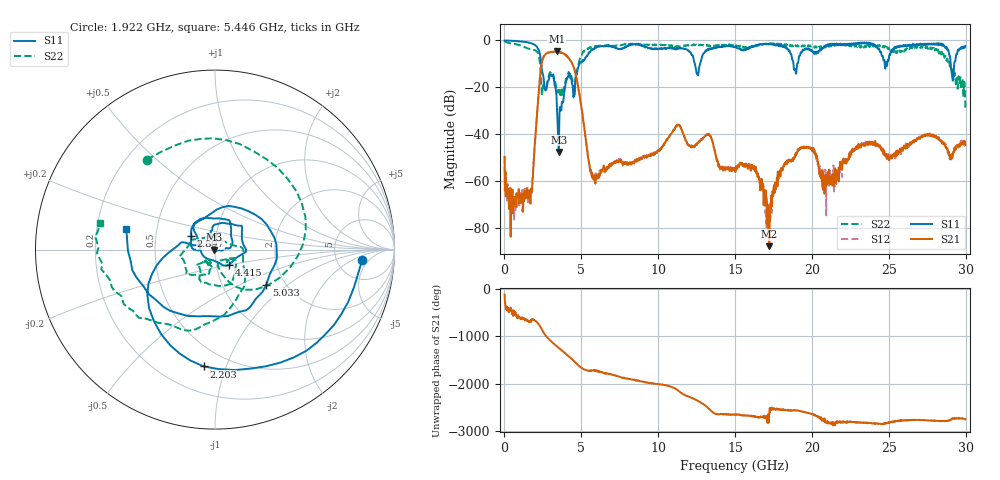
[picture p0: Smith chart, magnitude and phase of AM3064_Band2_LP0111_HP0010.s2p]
# Hz S DB R 50.0
!freq dBS11 angS11 dBS21 angS21 dBS12 angS12 dBS22 angS22
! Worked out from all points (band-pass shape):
!   1600 points, 10 MHz to 29.98 GHz, reference 50 ohm
!   highest |S21| = -4.74 dB at 3.403 GHz (marker M1); lowest = -87.9 dB at 17.22 GHz (marker M2)
!   |S21| within 3 dB of the highest: 2.503 GHz to 4.196 GHz (1.692 GHz wide, 50.5 % of centre)
!   lowest |S11| = -47.7 dB at 3.534 GHz (marker M3), VSWR 1.01, Z = 49.6 - j0.0628 ohm
!   |S11| at or under -10 dB: 2.398 GHz to 4.876 GHz (2.478 GHz wide, 68.1 % of centre); 12.38 GHz to 12.73 GHz (342.2 MHz wide, 2.73 % of centre); 18.8 GHz to 19.05 GHz (251.1 MHz wide, 1.33 % of centre)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
!   |S22| runs from -29.2 to -0.2 dB; largest |S21 - S12| = 0.016
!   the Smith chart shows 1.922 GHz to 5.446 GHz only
!   S11 on the Smith chart (normalised r, x): 1.922 GHz: 8.98, -3.34; 2.203 GHz: 0.37, -0.84; 2.897 GHz: 0.76, +0.12; 4.415 GHz: 1.15, -0.20; 5.033 GHz: 1.60, -0.72; 5.446 GHz: 0.33, +0.10
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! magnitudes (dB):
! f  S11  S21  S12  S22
! 10 MHz  0.0  -49.7  -49.9  -0.2
! 647.3 MHz  -0.3  -69.3  -71.7  -1.5
! 1.659 GHz  -1.1  -64.1  -67.7  -3.7
! 1.922 GHz  -1.7  -49.7  -49.2  -4.0
! 2.203 GHz  -3.7  -24.3  -24.3  -5.7
! 2.897 GHz  -16.3  -5.2  -5.1  -14.7
! 3.403 GHz  -26.5  -4.7  -4.9  -21.3
! 3.534 GHz  -47.7  -4.9  -4.9  -21.6
! 4.415 GHz  -18.8  -10.1  -10.0  -16.6
! 5.015 GHz  -9.5  -29.0  -29.0  -6.3
! 5.033 GHz  -9.2  -29.8  -29.6  -6.2
! 5.446 GHz  -5.9  -50.2  -49.7  -3.7
! 10 GHz  -3.6  -47.3  -47.0  -2.0
! 11.31 GHz  -3.2  -36.2  -36.0  -2.6
! 15 GHz  -2.6  -54.9  -54.6  -2.1
! 17.22 GHz  -1.4  -87.9  -75.4  -1.5
! 18.14 GHz  -2.9  -54.1  -53.5  -1.9
! 19.99 GHz  -4.3  -46.4  -47.0  -2.2
! 20.87 GHz  -2.3  -60.8  -55.2  -3.1
! 25 GHz  -8.0  -49.8  -51.1  -3.1
! 28.31 GHz  -1.7  -42.6  -42.7  -4.7
! 29.98 GHz  -2.4  -44.8  -45.2  -29.2
